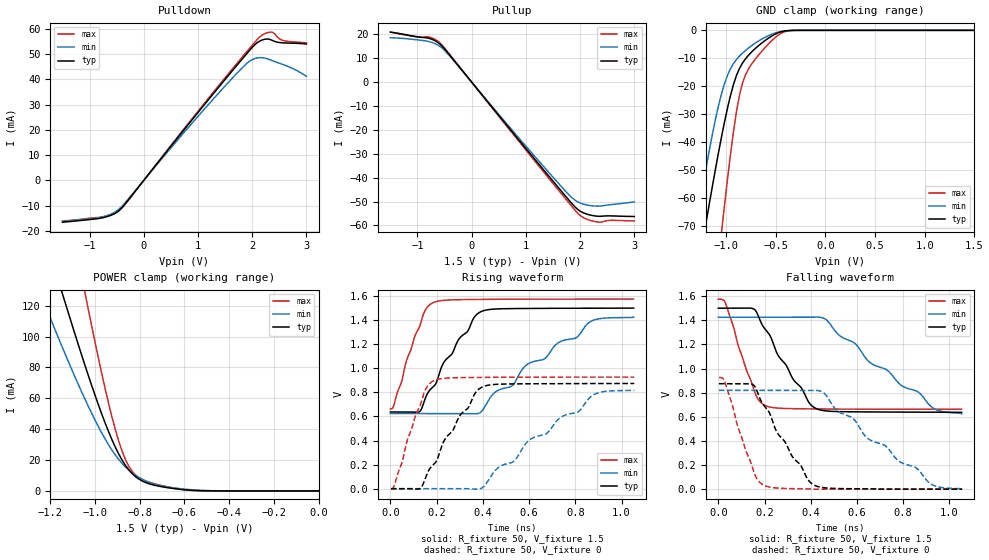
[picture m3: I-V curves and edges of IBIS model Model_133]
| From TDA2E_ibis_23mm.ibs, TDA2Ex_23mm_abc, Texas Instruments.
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| Model based on original model for DDR_SEIOPB_H
|   Sub model SR111_DRV34_1P5
[model]   Model_133
|[Description]  [1.5V-I/O-X-X]
|   , ,
|[Input Load]
|[Output Drive]
|Voltage   1.5V
|Mode   I/O
Model_type   I/O
Polarity   Non-Inverting
Enable   Active-Low
Vinl =  0.65
Vinh =  0.85
Cref =  15.0000pF
Rref =  100.0000M
Vref =  0V
Vmeas =  0.75
C_comp   2p   2p   2p
[Model Spec]
Vinl   0.65   0.6125   0.6875
Vinh   0.85   0.8125   0.8875
[Receiver Thresholds]
Tslew_ac = 0.5n
Vth= 0.75
Vth_max= 0.7875
Vth_min= 0.675
Vinh_ac= 0.175
Vinh_dc= 0.1
Vinl_ac= -0.175
Vinl_dc= -0.1
[Temperature Range]   25   125   -40
[Voltage Range]   1.5   1.425   1.575
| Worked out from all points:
|   slope of the pulldown table from 0 to 0.225 V, typ, clamps not added: 36.8 ohm
|   slope of the pullup table from 0 to 0.225 V, typ, clamps not added: 35.8 ohm
|   GND clamp passes 1 mA (typ) near -0.48 V on its own axis
|   POWER clamp passes 1 mA (typ) near -0.62 V on its own axis
|   rising waveform, R_fixture 50, V_fixture 1.5: 20-80 % time 173ps typ, 368ps min, 93.9ps max; typ from 0.637 V to 1.5 V
|   rising waveform, R_fixture 50, V_fixture 0: 20-80 % time 170ps typ, 362ps min, 92.8ps max; typ from 0 V to 0.874 V
|   falling waveform, R_fixture 50, V_fixture 1.5: 20-80 % time 166ps typ, 346ps min, 92.9ps max; typ from 1.5 V to 0.637 V
|   falling waveform, R_fixture 50, V_fixture 0: 20-80 % time 168ps typ, 352ps min, 93.2ps max; typ from 0.874 V to 0 V
[POWER_clamp]
-1.5V     302.8mA    223.9mA    484.4mA
-1.242V   174.3mA    127.3mA    279.1mA
-1.136V   123.3mA    89.68mA    196.8mA
-1.045V   81.65mA    59.62mA    128.8mA
-1.03V    75mA       54.92mA    117.8mA
-939.4mV  38.44mA    29.91mA    56.84mA
-893.9mV  23.93mA    20.41mA    32.31mA
-848.5mV  13.61mA    13.43mA    15.91mA
-803mV    7.623mA    8.663mA    8.564mA
-712.1mV  3.022mA    3.561mA    3.877mA
-575.8mV  470.5uA    872uA      449uA
0V        112.6nA    435.6nA    613.8nA
[Pulldown]
-1.5V     -16.54mA   -16.32mA   -16.11mA
-727.3mV  -14.62mA   -14.26mA   -14.29mA
-545.5mV  -13.24mA   -12.72mA   -13.05mA
-409.1mV  -10.94mA   -10.36mA   -11.07mA
1.227V    32.84mA    30.87mA    33.41mA
1.818V    48.09mA    44.61mA    48.84mA
2V        52.62mA    47.82mA    53.46mA
2.182V    55.55mA    48.58mA    57.5mA
2.273V    55.99mA    48.2mA     58.42mA
2.364V    55.5mA     47.46mA    58.71mA
2.545V    54.48mA    46.06mA    55.55mA
3V        54mA       41.23mA    54.49mA
[Pullup]
-1.5V     20.96mA    18.6mA     20.95mA
-1V       19mA       17.69mA    18.93mA
-772.7mV  18.26mA    16.89mA    18.84mA
-590.9mV  16.04mA    15.07mA    16.54mA
-409.1mV  11.43mA    11.07mA    11.7mA
1.409V    -38.97mA   -37.46mA   -39.88mA
1.773V    -48.83mA   -46.66mA   -49.96mA
1.909V    -52.33mA   -49.44mA   -53.68mA
2.045V    -54.57mA   -50.97mA   -56.55mA
2.273V    -56.03mA   -51.89mA   -58.38mA
2.591V    -56.03mA   -51.23mA   -57.86mA
3V        -56.26mA   -50.14mA   -58.12mA
[GND_clamp]
-1.5V     -133.6mA   -115.7mA   -234.3mA
-1.288V   -87.29mA   -67.59mA   -156.8mA
-1.197V   -68.11mA   -48.64mA   -124.4mA
-1.045V   -38.25mA   -22.77mA   -72.51mA
-1.015V   -32.88mA   -19.1mA    -62.74mA
-954.5mV  -23.3mA    -13.72mA   -44.4mA
-863.6mV  -13.6mA    -9.192mA   -23.11mA
-803mV    -10.18mA   -7.193mA   -15.89mA
-681.8mV  -5.771mA   -4.027mA   -9.287mA
-500mV    -1.264mA   -914.7uA   -2.429mA
-348.5mV  -52.39uA   -75.11uA   -85.87uA
1.5V      112.6nA    528.1nA    514.5nA
[Ramp]
dV/dt_f  0.5184208/0.16650507n 0.48157253/0.34697508n 0.54815265/93.048661p
dV/dt_r 0.52643212/0.17117935n 0.49371973/0.36366008n 0.55768225/93.202655p
R_load = 50
[Rising Waveform]
R_fixture = 50
V_fixture = 1.5
V_fixture_min = 1.425
V_fixture_max = 1.575
0s        637.3mV    624.3mV    663.3mV
125.3ps   639.4mV    624.2mV    1.342V
150.7ps   748.5mV    624.2mV    1.482V
184.8ps   845.7mV    624.3mV    1.545V
294.6ps   1.237V     624.1mV    1.57V
397.4ps   1.475V     648.4mV    1.572V
587.2ps   1.497V     1.025V     1.574V
806.7ps   1.499V     1.257V     1.575V
863ps     1.499V     1.385V     1.575V
1.053ns   1.5V       1.425V     1.575V
[Rising Waveform]
R_fixture = 50
V_fixture = 0
V_fixture_min = 0
V_fixture_max = 0
2.527ps   0V         0V         0V
17.3ps    0V         0V         28.41mV
129.3ps   0V         0V         692.7mV
155.4ps   108.7mV    0V         836.6mV
189.3ps   206mV      0V         898.3mV
298.9ps   602.4mV    0V         922.3mV
400.2ps   847mV      11.22mV    924.6mV
598.9ps   871.5mV    400.3mV    926.2mV
874.9ps   873.3mV    775mV      926.6mV
1.055ns   874.1mV    819mV      926.7mV
[Falling Waveform]
R_fixture = 50
V_fixture = 1.5
V_fixture_min = 1.425
V_fixture_max = 1.575
0s        1.5V       1.425V     1.575V
32.03ps   1.5V       1.425V     1.537V
151.3ps   1.495V     1.425V     840.6mV
203.7ps   1.324V     1.425V     692.6mV
323.2ps   913.4mV    1.425V     667.3mV
424.6ps   667mV      1.427V     664.8mV
465.6ps   648.6mV    1.406V     664.2mV
655ps     640mV      1.052V     662.8mV
928.1ps   638.2mV    673.7mV    662.4mV
1.053ns   637.3mV    624.3mV    662.3mV
[Falling Waveform]
R_fixture = 50
V_fixture = 0
V_fixture_min = 0
V_fixture_max = 0
2.527ps   874.1mV    819mV      926.7mV
29.11ps   874.2mV    819mV      886mV
147.9ps   868.5mV    819.1mV    177.5mV
198.6ps   690.9mV    819mV      31.08mV
319ps     273.7mV    818.8mV    4.462mV
421.2ps   27.92mV    819mV      0V
584ps     3.393mV    584.3mV    0V
645ps     2.456mV    423.3mV    0V
918.9ps   0V         44.12mV    0V
1.055ns   0V         0V         0V
